{attribute 'qualified_only'}
VAR_GLOBAL
	{attribute 'TcContextName' := 'PlcCommunication'}	
	g_stKL6831KL6841InData			 AT %I*	: ST_KL6831KL6841InData;
	{attribute 'TcContextName' := 'PlcCommunication'}	
	g_stKL6831KL6841OutData		 	 AT %Q*	: ST_KL6831KL6841OutData;
	g_stCommandBuffer						: ST_SMICommandBuffer;	
END_VAR
